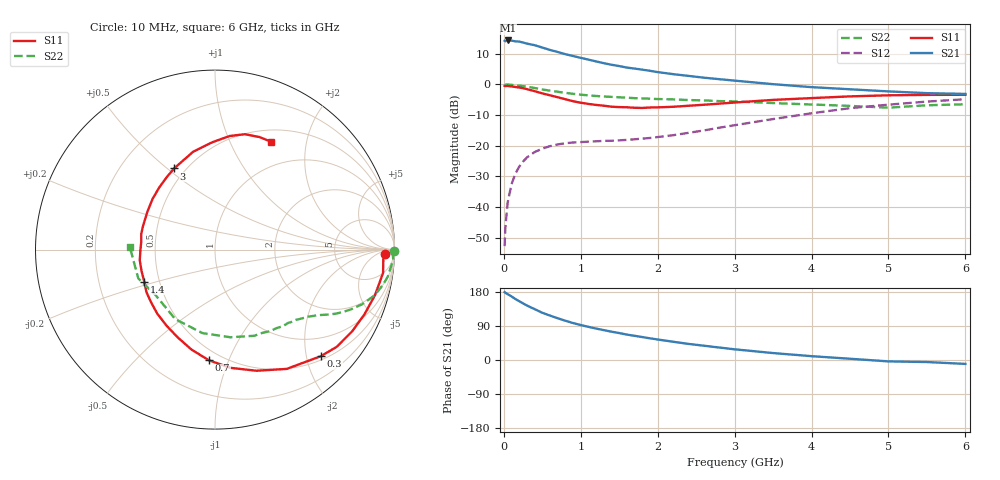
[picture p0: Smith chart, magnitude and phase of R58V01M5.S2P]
! SIEMENS Small Signal Semiconductors
! BFR183
! Si NPN RF Bipolar Junction Transistor in SOT23
! VCE = 8 V  IC = 1.5 mA
! Common Emitter S-Parameters:  May  1996
# GHz  S  MA  R  50
!  f  S11  S21  S12  S22
! GHz  MAG  ANG  MAG  ANG  MAG  ANG  MAG  ANG
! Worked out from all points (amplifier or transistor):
!   36 points, 10 MHz to 6 GHz, reference 50 ohm
!   highest |S21| = 14.3 dB at 50 MHz (marker M1)
!   |S21| within 3 dB of that: start of sweep to 587.7 MHz
!   unconditionally stable (mu >= 1): 1.537 GHz to 2.899 GHz
!   at 250 MHz: K = 0.19, MSG = 19.4 dB, |S12| = -25.2 dB
!   at 1.4 GHz: K = 0.94, MSG = 12.4 dB, |S12| = -18.4 dB
!   at 6 GHz: K = 0.91, MSG = 0.9 dB, |S12| = -4.8 dB
!   S11 on the Smith chart (normalised r, x): 10 MHz: 28, -14; 300 MHz: 0.57, -2.29; 700 MHz: 0.43, -0.85; 1.4 GHz: 0.41, -0.18; 3 GHz: 0.43, +0.53; 6 GHz: 0.65, +1.44
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0.01  0.9448 -1.6  5.155 179.1  0.0023 88.9  0.9962 -0.5
0.02  0.9394 -3.3  5.06 177.4  0.0047 88.8  0.99 -1.2
0.05  0.9454 -7.9  5.21 173.8  0.0119 84.0  0.9942 -3.1
0.1  0.9268 -15.9  5.18 167.8  0.0236 80.9  0.9836 -6.0
0.15  0.9075 -23.4  5.038 160.9  0.0349 76.3  0.9743 -8.9
0.2  0.8896 -30.8  4.999 155.1  0.0456 72.4  0.9569 -11.7
0.3  0.8376 -45.1  4.629 143.8  0.0644 64.6  0.9193 -16.5
0.4  0.7755 -59.0  4.365 134.3  0.0788 58.1  0.8744 -20.4
0.5  0.7134 -71.1  3.989 124.6  0.0896 52.6  0.828 -23.7
0.6  0.6645 -82.5  3.648 117.2  0.0984 48.2  0.7901 -26.2
0.7  0.6177 -93.1  3.379 110.2  0.105 45.1  0.7588 -28.1
0.8  0.5732 -103.0  3.11 103.6  0.1098 42.3  0.7284 -29.8
0.9  0.5316 -113.0  2.905 97.5  0.1129 40.7  0.702 -31.2
1.1  0.4805 -132.0  2.537 87.5  0.1166 39.0  0.6621 -33.9
1.4  0.4326 -155.7  2.09 74.7  0.1205 39.1  0.6261 -37.4
1.8  0.4132 174.1  1.739 60.5  0.1307 44.4  0.5909 -42.1
2.2  0.4316 150.9  1.471 48.2  0.1483 50.1  0.5704 -48.4
3  0.5063 116.8  1.153 28.2  0.216 55.4  0.5279 -65.4
3.5  0.5589 102.5  1.009 18.3  0.2722 53.3  0.496 -80.0
4.5  0.6379 82.7  0.833 3.3  0.4098 41.9  0.4462 -119.7
5.5  0.6743 68.4  0.72 -5.4  0.5248 26.7  0.4566 -159.4
6  0.6777 62.4  0.7 -10.3  0.5728 17.1  0.4744 178.3
